FUNCTION_BLOCK FB52
TITLE =Get Movement State
//*****************************************************************************
//* maxon motor ag
//* R&D
//* all rights reserved
//*****************************************************************************
//* Summary:  Read if the drive has reached the target
//*
//* Remarks:
//*
//* Created under: STEP7 REV5.2+SP1
//*****************************************************************************
//* History:
//* 19.05.2004 | INA   first release
//*
//*
//*****************************************************************************
//

AUTHOR:INA
FAMILY:MotionIn
NAME:GetMovSt
VERSION:00.01


VAR_INPUT

Read : BOOL //A rising edge start the command

  NodeID : BYTE //Adress of the maxon device

END_VAR
VAR_OUTPUT
  Done : BOOL //Data valid flag is TRUE if data were available

  Err : BOOL //Error flag is TRUE if an Error has occured, see ErrNo for more details

  ErrNo : DINT //Contains detailed error information

  TargetReached : BOOL //The drive has reached the target

END_VAR
VAR
  xEdgeMerker : BOOL //Edge Merker

  xEdgeFlag : BOOL //Edge Flag

  xStep : INT
  xControlword : INT
END_VAR

BEGIN

NETWORK
TITLE = Activate the service function
//

// SDO Read "Get Movement State"

       U    #Read
       FP   #xEdgeFlag                   // recognize a positiv edge of the Read signal
       =    #xEdgeMerker                 // and set the xEdgeMerker for one cycle to true

       L    #xStep
       L    0
       ==I
       U    #xEdgeMerker
       SPB  nstp                         // iStep = 1 -> fnc1

       L    #xStep                       // jump list
       SPL  List
       SPA  rdef
       SPA  fnc1
       SPA  fncE
List  :SPA  rdef

rdef  :NOP  0
       R    #Done                        // reset Done
       R    #Err                         // reset Error
       L    0
       T    #xStep                       // iStep = 0
       SPA  end

fnc1  :NOP  0
       CALL FC1
         NodeID:=#NodeID
         Index:=DW#16#00006041
         SubIndex:=DW#16#00000000
         RET_VAL:=#Done
         Err:=#Err
         ErrNo:=#ErrNo

       S    #Done

       L    DB219.DBD10
       UW   W#16#0400
       T    #xControlword

       L    #xControlword
       L    W#16#0400
       ==I
       SPB  tdis
       SPA  fdis

tdis  :NOP  0
       S    #TargetReached               // set Target Reached
       SPA  fncE

fdis  :NOP  0
       R    #TargetReached               // reset Target Reached
       SPA  fncE

fncE  :NOP  0
       L    0
       T    #xStep
       SPA  end

nstp  :NOP  0
       L    #xStep
       INC            1
       T    #xStep

end   :NOP  0
END_FUNCTION_BLOCK
